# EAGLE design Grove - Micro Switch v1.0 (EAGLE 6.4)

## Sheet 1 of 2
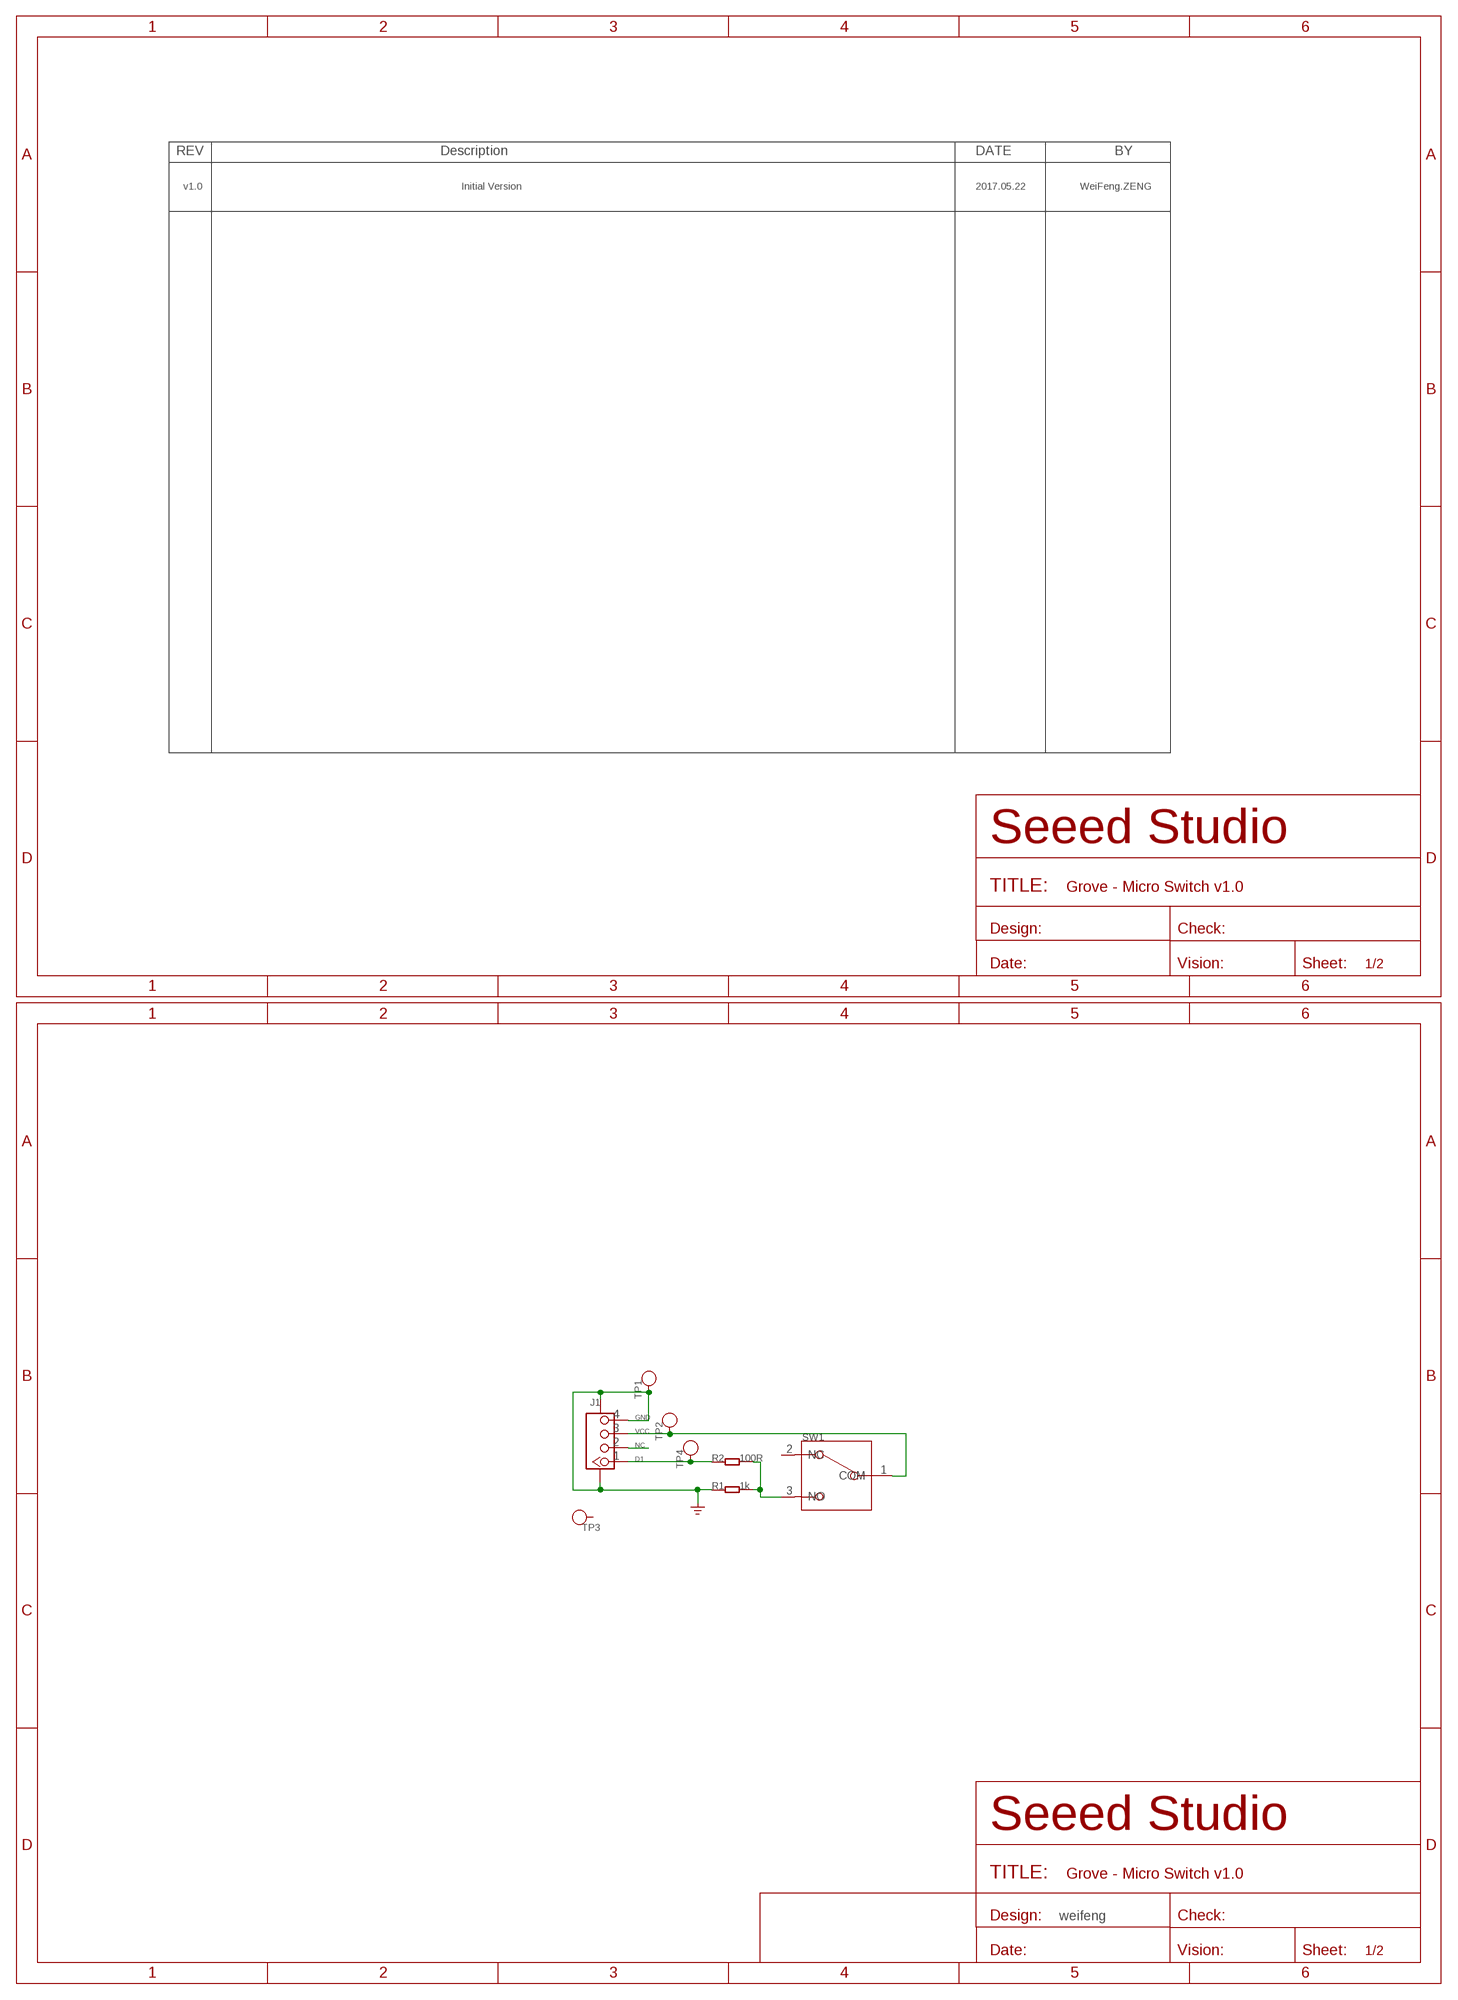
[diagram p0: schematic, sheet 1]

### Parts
J1  GROVE-CONNECTOR-SMD'90D'  [HW4-SMD-2.0-90D]
R1  1k  RES-0603  [R0603]
R2  100R  RES-0603  [R0603]
SW1  SWITCH-ZW12-N  [SW3-19.8X6.3X10.6MM]
TP1  TEST-POINT'4545'  [TP-D45MIL]
TP2  TEST-POINT'4545'  [TP-D45MIL]
TP3  TEST-POINT'4545'  [TP-D45MIL]
TP4  TEST-POINT'4545'  [TP-D45MIL]

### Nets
D1: J1.1 R2.1 TP4.T
GND: J1.4 J1.SS1 J1.SS2 R1.1 TP1.T ; supply symbol labelled GND_POWER
N$5: R1.2 R2.2 SW1.3(NO)
NC: J1.2
VCC: J1.3 SW1.1(COM) TP2.T
Unconnected: SW1.2(NC) TP3.T

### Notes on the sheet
- v1.0 | Initial Version | 2017.05.22 | WeiFeng.ZENG
- weifeng

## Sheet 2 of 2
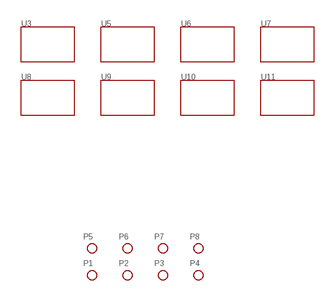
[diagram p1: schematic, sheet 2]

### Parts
P1  PAD-MARK  [ROUND-MARK-1.0]
P2  PAD-MARK  [ROUND-MARK-1.0]
P3  PAD-MARK  [ROUND-MARK-1.0]
P4  PAD-MARK  [ROUND-MARK-1.0]
P5  PAD-MARK  [ROUND-MARK-1.0]
P6  PAD-MARK  [ROUND-MARK-1.0]
P7  PAD-MARK  [ROUND-MARK-1.0]
P8  PAD-MARK  [ROUND-MARK-1.0]
U3  TWIG'2U'  [GROVE-TEST-PLATFORM]
U5  TWIG'2U'  [GROVE-TEST-PLATFORM]
U6  TWIG'2U'  [GROVE-TEST-PLATFORM]
U7  TWIG'2U'  [GROVE-TEST-PLATFORM]
U8  TWIG'2U'  [GROVE-TEST-PLATFORM]
U9  TWIG'2U'  [GROVE-TEST-PLATFORM]
U10  TWIG'2U'  [GROVE-TEST-PLATFORM]
U11  TWIG'2U'  [GROVE-TEST-PLATFORM]

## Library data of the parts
J1 = Connector-new:GROVE-CONNECTOR-SMD: 4P-SMD-2.0:320110030;4P-SMD-2.0-90D:320110032
P1-P8 = Discrete:PAD-MARK; PARTNO: DNP
R1 R2 = discrete-new:RES
SW1 = discrete-new:SWITCH-ZW12-N
TP1-TP4 = discrete-new:TEST-POINT; PARTNO: DNP
U3 U5-U11 = template:TWIG

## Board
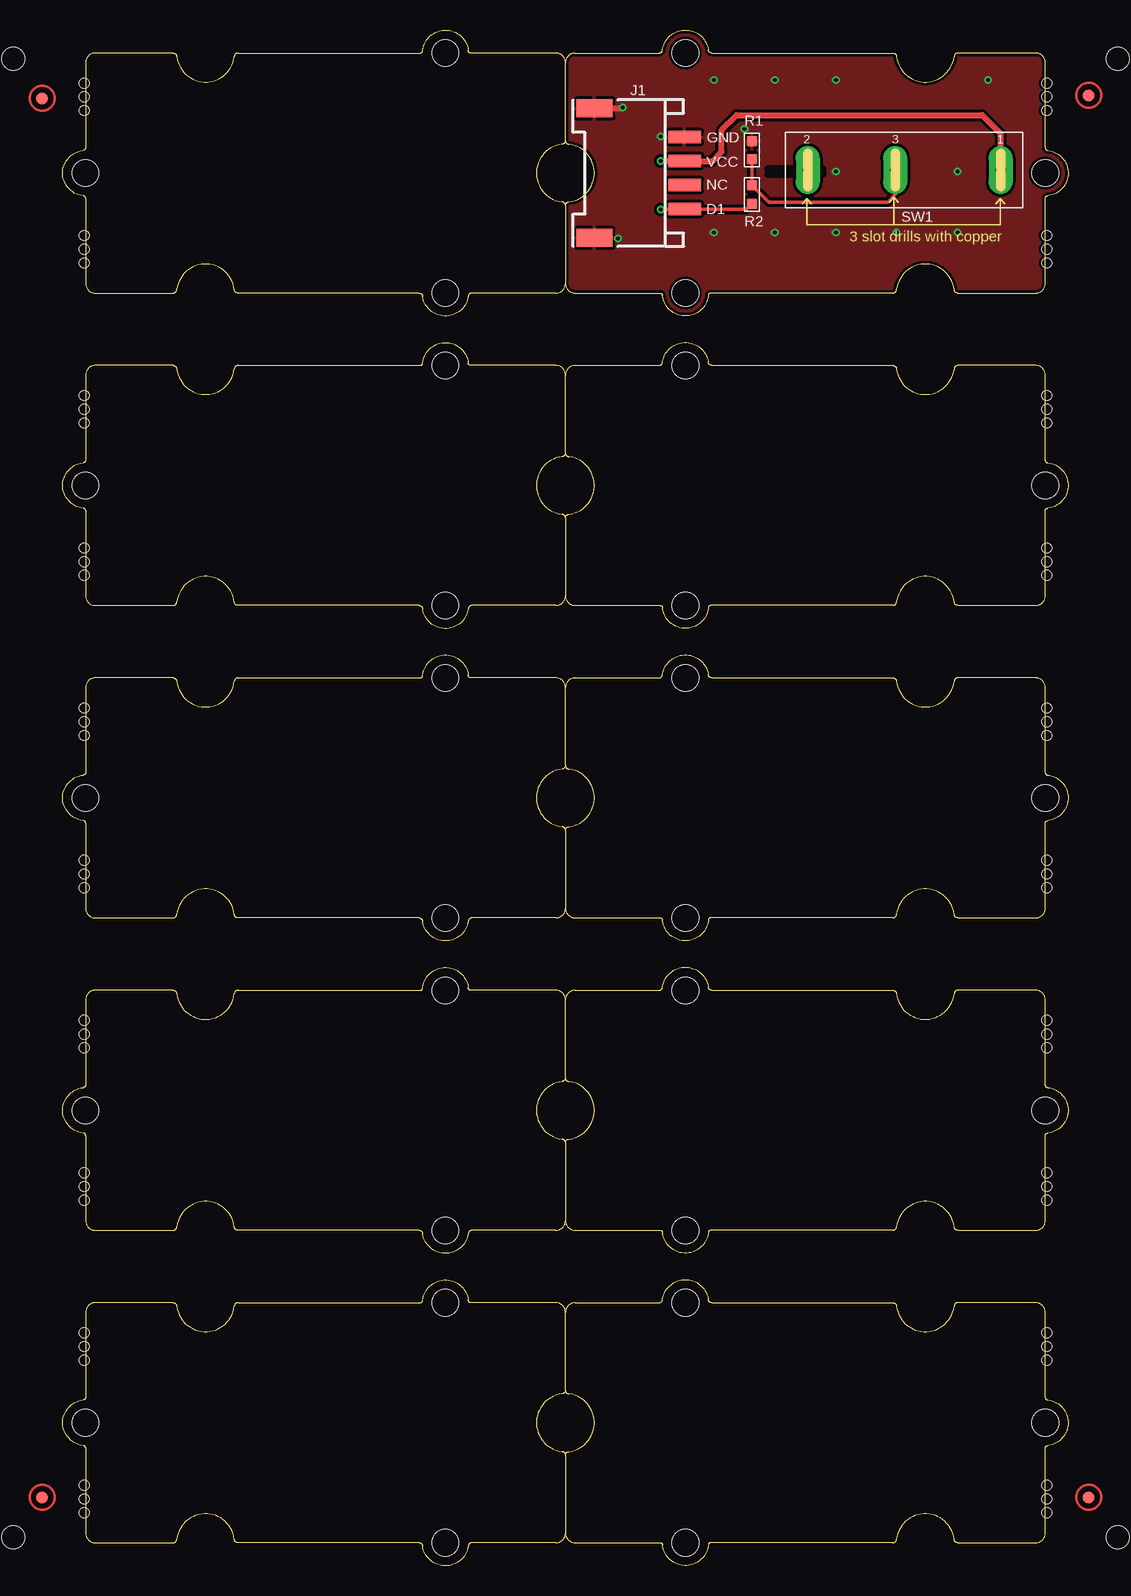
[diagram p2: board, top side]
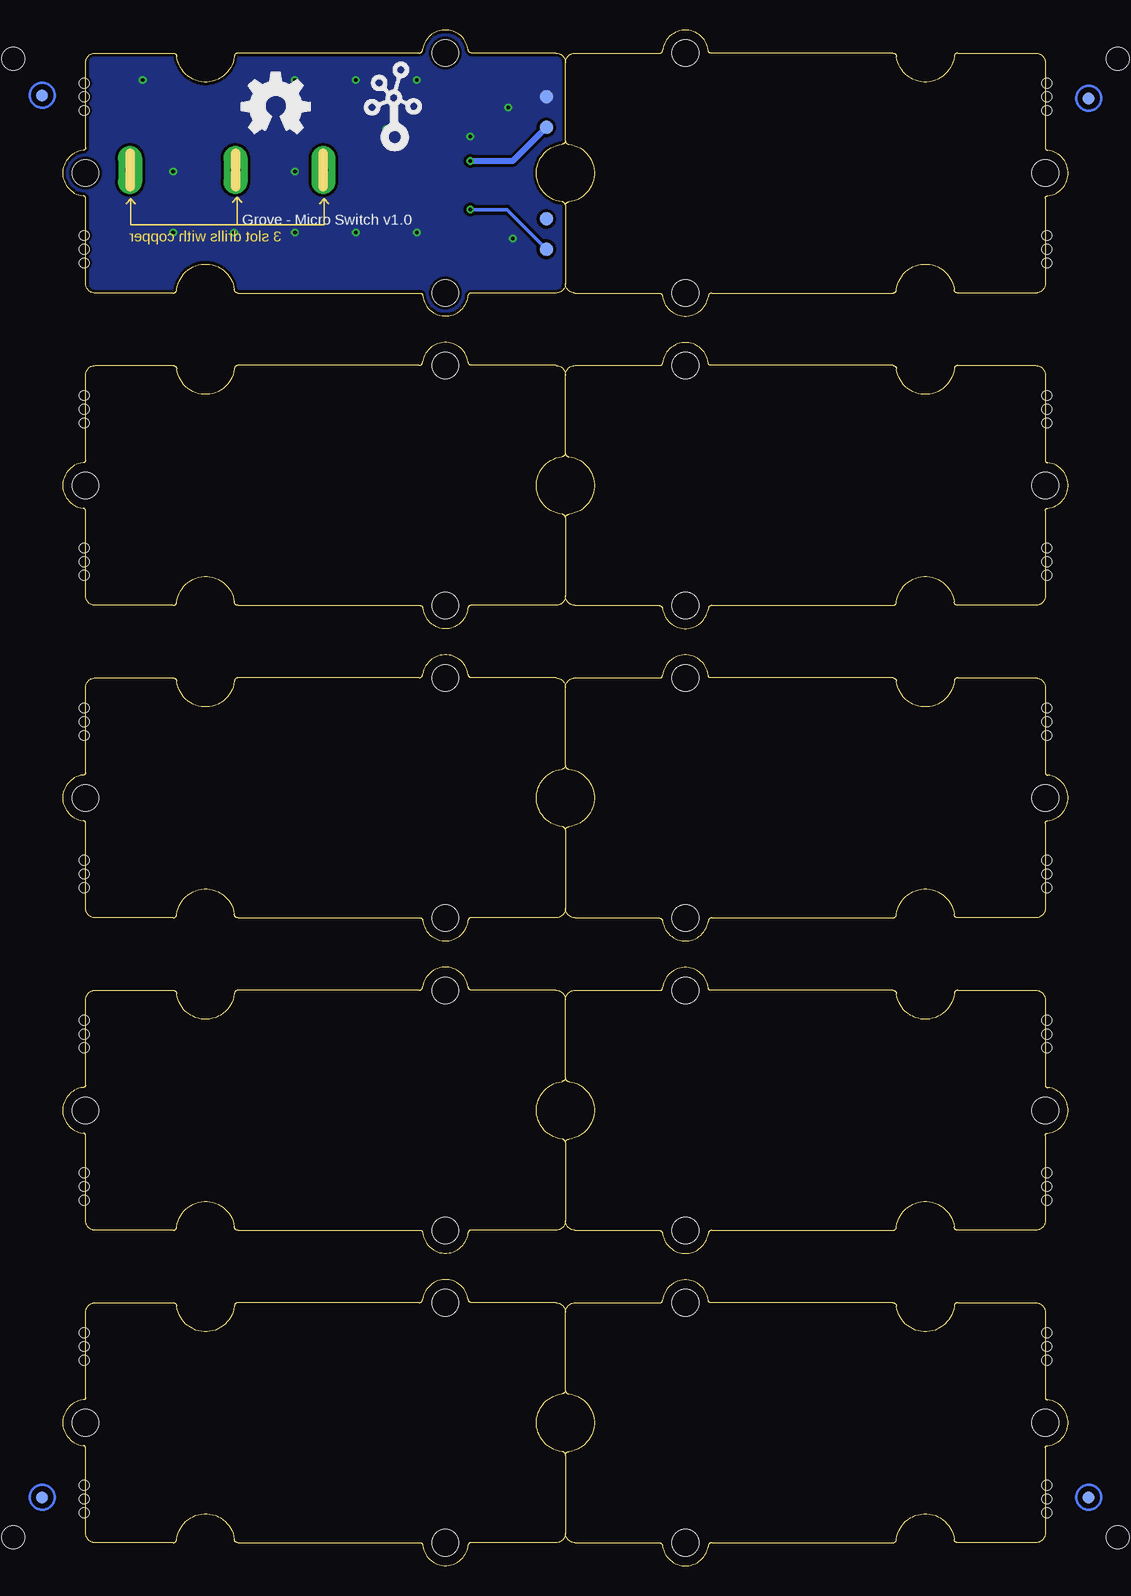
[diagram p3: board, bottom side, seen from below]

Size 83.82 x 127.98 mm. Coordinates in mm from the lower left corner, seen from the top.
Copper layers (1*16): Top 0.035mm / dielectric 1.5mm / Bottom 0.035mm
Design rules "SeeedStudio_2layer_DRU_no_angle_20140221 *": minimum track width 6mil, minimum drill 12mil, track to track 6mil, track to pad 6mil, pad to pad 6mil, via to via 6mil, smd to smd 0mil, copper to edge 10mil, drill to drill 10mil, minimum pad ring 10mil, minimum via ring 6mil, stop-mask expansion 2mil, vias tented up to drill 100mil, thermal gap 10mil
Holes 0.8 mm at 1.78,123.55 1.78,121.27 1.78,122.41 1.78,110.85 1.78,108.57 1.78,109.71 1.78,97.52 1.78,95.23 1.78,96.38 1.78,84.82 1.78,82.53 1.78,83.68 1.78,71.48 1.78,69.2 1.78,70.34 1.78,58.78 1.78,56.5 1.78,57.64 1.78,45.45 1.78,43.16 1.78,44.31 1.78,32.75 1.78,30.46 1.78,31.61 1.78,19.41 1.78,17.13 1.78,18.27 1.78,6.71 1.78,4.43 1.78,5.57 82.04,121.27 82.04,123.55 82.04,122.41 82.04,108.57 82.04,110.85 82.04,109.71 82.04,95.23 82.04,97.52 82.04,96.38 82.04,82.53 82.04,84.82 82.04,83.68 82.04,69.2 82.04,71.48 82.04,70.34 82.04,56.5 82.04,58.78 82.04,57.64 82.04,43.16 82.04,45.45 82.04,44.31 82.04,30.46 82.04,32.75 82.04,31.61 82.04,17.13 82.04,19.41 82.04,18.27 82.04,4.43 82.04,6.71 82.04,5.57
Holes 1.91 mm at -4.13,2.4 87.95,2.4 87.95,125.59 -4.13,125.59
tRestrict: area 58.7,115.9 to 63.4,116.4

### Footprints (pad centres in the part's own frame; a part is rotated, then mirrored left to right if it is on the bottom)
HW4-SMD-2.0-90D = smd 1.01 x 2.74: 1 -3,-0.1; 2 -1,-0.1; 3 1,-0.1; 4 3,-0.1 | smd 1.5 x 3: SS1 -5.4,7.4; SS2 5.4,7.4
ROUND-MARK-1.0 = smd 1.016 x 1.016: P$1 0,0
R0603 = smd 0.889 x 0.889: 1 0,0.762; 2 0,-0.762
SW3-19.8X6.3X10.6MM = drill 0.8 pad 2 long: 1 -8.8,0; 2 7.3,0; 3 0,0
TP-D45MIL = smd 1.143 x 1.143: T 0,0
GROVE-TEST-PLATFORM = hole 2.2: -10,-10; -10,10; 20,0

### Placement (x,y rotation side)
J1  51.75,116.06 90 top
P1  -1.71,5.7 0 top
P2  85.54,5.7 0 top
P3  -1.71,122.28 0 top
P4  85.54,122.54 0 top
P5  -1.71,5.7 0 bottom
P6  85.54,5.7 0 bottom
P7  85.54,122.54 0 bottom
P8  -1.71,122.28 0 bottom
R1  57.47,117.97 0 top
R2  57.47,114.28 180 top
SW1  69.41,116.32 180 top
TP1  43.5,122.41 0 bottom
TP2  43.5,119.87 0 bottom
TP3  43.5,112.25 0 bottom
TP4  43.5,109.71 0 bottom
U3  61.91,37.96 0 top
U5  21.91,37.96 180 top
U6  61.91,63.99 0 top
U7  21.91,63.99 180 top
U8  61.91,90.03 0 top
U9  21.91,90.03 180 top
U10  21.91,116.06 180 top
U11  61.91,116.06 0 top
U12  [GROVE-TEST-PLATFORM]  61.91,11.92 0 top
U13  [GROVE-TEST-PLATFORM]  21.91,11.92 180 top
U$7  [OSHW_FILLX200_NOTEXT]  68.9,119.36 0 bottom
U$8  [TWIGLOGO]  56.2,118.86 0 bottom

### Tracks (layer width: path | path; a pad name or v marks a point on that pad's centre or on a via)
D1  (via drill 0.3 pad 0.64)
  Top 0.305: R2.1 57.01,113.06 J1.1 49.9,113.06 v49.85,113.01
  Bottom 0.305: v49.85,113.01 46.8,113.01 TP4.T
GND  (via drill 0.3 pad 0.64)
  Top 0.508: J1.SS2 46.61,121.46 v46.67,121.52
  other vias: 49.85,119.11 56.83,119.74 46.29,110.6 54.29,123.81 59.37,123.81 64.45,123.81 64.45,116.19 64.45,111.11 59.37,111.11 54.29,111.11 69.53,111.11 74.61,111.11 74.61,116.19 77.15,123.81
  pour Top (isolate 0.254): 41.59,128.25 84.14,128.25 84.14,104.12 41.59,104.12
  pour Bottom (isolate 0.254): 41.59,128.25 84.14,128.25 84.14,104.12 41.59,104.12
N$5
  Top 0.305: R1.2 R2.2 58.87,113.65 68.77,113.65 69.41,114.28 SW1.3
VCC  (via drill 0.3 pad 0.64)
  Top 0.508: v49.85,117.08 49.86,117.06 J1.3 54.15,117.06 54.93,117.84 54.93,119.62 56.2,120.89 76.65,120.89 78.21,119.33 SW1.1
  Bottom 0.508: v49.85,117.08 46.29,117.08 TP2.T

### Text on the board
tNames: GND | VCC | NC | D1
bNames: Grove - Micro Switch v1.0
